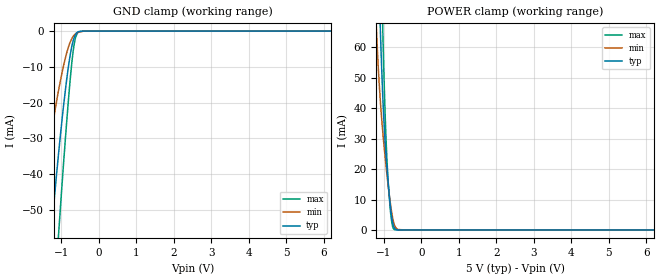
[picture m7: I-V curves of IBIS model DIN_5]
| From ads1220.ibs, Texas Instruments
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[Model]   DIN_5
Model_type   Input
Vinl = 1.35
Vinh = 3.85
|   typ   min   max
|   (nom PVT)   (Fast PVT)   (slow PVT)
C_comp   5.766p   5.315p   6.202p
| Where   nom PVT is  Nominal Process, 5V, 27C
|   Fast PVT is Strong Process, 5.5V, -40C
|   Slow PVT is Weak Process, 4.5V, 125C
[Voltage Range]   5   4.5   5.5
[Temperature Range]   27   125   -40
[Power Clamp Reference]   5   4.5   5.5
[GND Clamp Reference]   0   0   0
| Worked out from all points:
|   GND clamp passes 1 mA (typ) near -0.62 V on its own axis
|   POWER clamp passes 1 mA (typ) near -0.73 V on its own axis
[GND Clamp]
|   Voltage   I(typ)   I(min)   I(max)
-5V       -582.7mA   -403.4mA   -706.6mA
-1.67V    -107.2mA   -58.7mA    -153.4mA
-1.52V    -87.57mA   -46.72mA   -128.6mA
-1.385V   -70.46mA   -36.65mA   -106.4mA
-1.25V    -54.09mA   -27.34mA   -84.55mA
-1.1V     -37.08mA   -18.05mA   -60.87mA
-1.04V    -30.72mA   -14.69mA   -51.69mA
-860mV    -13.79mA   -6.22mA    -25.77mA
-725mV    -4.553mA   -2.204mA   -9.351mA
-635mV    -1.235mA   -878.9uA   -2.473mA
-545mV    -175.3uA   -299.2uA   -286.6uA
10V       0A         0A         0A
[POWER Clamp]
|   Voltage   I(typ)   I(min)   I(max)
-5V       2.22A      1.727A     2.719A
-1.25V    135.8mA    81.33mA    194.5mA
-1.19V    107.4mA    63.81mA    157.5mA
-1.115V   74.62mA    46.48mA    113mA
-1.085V   62.89mA    40.99mA    95.95mA
-1.04V    47.51mA    33.91mA    71.82mA
-1.025V   43.07mA    31.77mA    64.29mA
-950mV    25.97mA    22.11mA    32.82mA
-890mV    16.26mA    15.23mA    17.13mA
-800mV    5.229mA    6.538mA    3.559mA
-710mV    466.3uA    1.412mA    95.19uA
10V       0A         0A         0A
